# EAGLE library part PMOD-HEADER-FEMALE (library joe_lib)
FEMALE HEADER
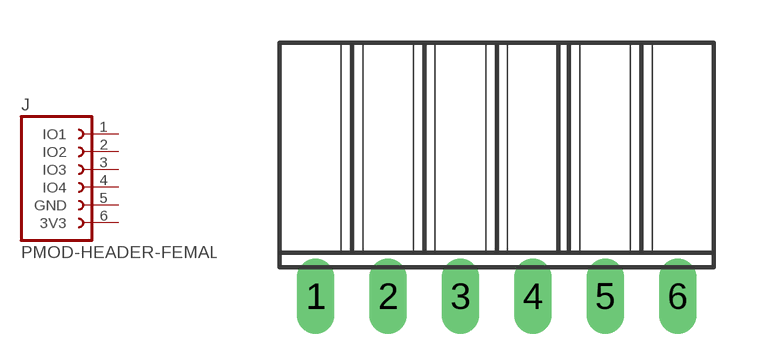
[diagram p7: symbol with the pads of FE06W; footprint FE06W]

Designator prefix J

## PMOD-HEADER-FEMALE (OC_FARNELL: unknown; OC_NEWARK: unknown)  [FE06W]
1  IO1
2  IO2
3  IO3
4  IO4
5  GND  pwr
6  3V3  pwr

## Footprint FE06W (pad centres in mm)
FEMALE HEADER
drill 0.813 long: 1 -6.35,0; 2 -3.81,0; 3 -1.27,0; 4 1.27,0; 5 3.81,0; 6 6.35,0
